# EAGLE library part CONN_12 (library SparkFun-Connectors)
Multi connection point. Often used as Generic Header-pin footprint for 0.1 inch spaced/style header connections On any of the 0.1 inch spaced packages, you can populate with these: Break Away Headers - Straight (PRT-00116) Break Away Male Headers - Right Angle (PRT-00553) Female Headers (PRT-00115) Break Away Headers - Machine Pin (PRT-00117) Break Away Female Headers - Swiss Machine Pin (PRT-00743) For SCREWTERMINALS and SPRING TERMINALS visit here: Screw Terimnals on SparkFun.com (5mm/3.5mm/2.54mm spacing) This device is also useful as a general connection point to wire up your design to another part of your project. Our various solder wires solder well into these plated through hole pads. Hook-Up Wire - Assortment (Stranded, 22 AWG) (PRT-11375) Hook-Up Wire - Assortment (Solid Core, 22 AWG) (PRT-11367) View the entire wire category on our website here Special notes: Molex polarized connector foot print use with SKU : PRT-08231 with associated crimp pins and housings. 1MM SMD Version SKU: PRT-10208 NOTES ON THE VARIANTS LOCK and LOCK_LONGPADS... This footprint was designed to help hold the alignment of a through-hole component (i.e. 6-pin header) while soldering it into place. You may notice that each hole has been shifted either up or down by 0.005 of an inch from it's more standard position (which is a perfectly straight line). This slight alteration caused the pins (the squares in the middle) to touch the edges of the holes. Because they are alternating, it causes a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
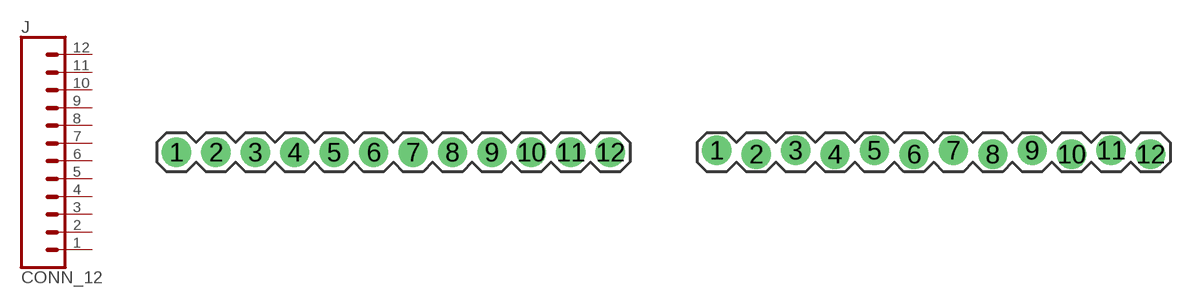
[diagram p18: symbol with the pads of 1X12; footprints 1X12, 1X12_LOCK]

Designator prefix J

## CONN_12  [1X12]
1  1  pas
2  2  pas
3  3  pas
4  4  pas
5  5  pas
6  6  pas
7  7  pas
8  8  pas
9  9  pas
10  10  pas
11  11  pas
12  12  pas

## CONN_12LOCK  [1X12_LOCK]
Pads as for 1X12

## CONN_12LOCK_LONGPADS  [1X12_LOCK_LONGPADS]
Pads as for 1X12

## CONN_12MACHINE-PIN_LOCK (PROD_ID: CONN-09704)  [1X12_MACHINE-PIN-HEADER_LOCK.004]
Pads as for 1X12

## CONN_12LONGPADS  [1X12_LONGPADS]
Pads as for 1X12

## CONN_12POGOPIN_HOLES_ONLY  [1X12_HOLES_ONLY]
Pads as for 1X12

## CONN_121X12_NO_SILK_KIT  [1X12_NO_SILK_KIT]
Pads as for 1X12

## CONN_12NO_SILK  [1X12_NO_SILK]
Pads as for 1X12

## CONN_12LOCK_NO_SILK  [1X12_LOCK_NO_SILK]
Pads as for 1X12

## CONN_12SM_SQ_NO_SILK  [1X12_SM_SQ_NOSILK]
Pads as for 1X12

## Footprint 1X12 (pad centres in mm)
Plated Through Hole -12 Pin Specifications: Pin count:12 Pin pitch:0.1" Example device(s): CONN_12
drill 1.016 pad 1.88: 1 0,0; 2 2.54,0; 3 5.08,0; 4 7.62,0; 5 10.16,0; 6 12.7,0; 7 15.24,0; 8 17.78,0; 9 20.32,0; 10 22.86,0; 11 25.4,0; 12 27.94,0

## Footprint 1X12_LOCK (pad centres in mm)
Plated Through Hole -12 Pin Locking Footprint Holes are offset 0.005", to hold pins in place during soldering. Specifications: Pin count:12 Pin pitch:0.1" Example device(s): CONN_12
drill 1.016 pad 1.88: 1 0,0.127; 2 2.54,-0.127; 3 5.08,0.127; 4 7.62,-0.127; 5 10.16,0.127; 6 12.7,-0.127; 7 15.24,0.127; 8 17.78,-0.127; 9 20.32,0.127; 10 22.86,-0.127; 11 25.4,0.127; 12 27.94,-0.127

## Footprint 1X12_LOCK_LONGPADS (pad centres in mm)
Plated Through Hole -12 Pin Locking Footprint with Long Pads Holes are offset 0.005", to hold pins in place during soldering. Specifications: Pin count:12 Pin pitch:0.1" Example device(s): CONN_12
drill 1.016 long: 1 0,0.127; 2 2.54,-0.127; 3 5.08,0.127; 4 7.62,-0.127; 5 10.16,0.127; 6 12.7,-0.127; 7 15.24,0.127; 8 17.78,-0.127; 9 20.32,0.127; 10 22.86,-0.127; 11 25.4,0.127; 12 27.94,-0.127

## Footprint 1X12_MACHINE-PIN-HEADER_LOCK.004 (pad centres in mm)
Plated Through Hole -12 Pin Machine Pin Headers Holes are offset 0.005", to hold pins in place during soldering. Specifications: Pin count:12 Pin pitch:0.1" Example device(s): CONN_12
drill 0.889 pad 1.88: 1 0,0.102; 2 2.54,-0.102; 3 5.08,0.102; 4 7.62,-0.102; 5 10.16,0.102; 6 12.7,-0.102; 7 15.24,0.102; 8 17.78,-0.102; 9 20.32,0.102; 10 22.86,-0.102; 11 25.4,0.102; 12 27.94,-0.102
